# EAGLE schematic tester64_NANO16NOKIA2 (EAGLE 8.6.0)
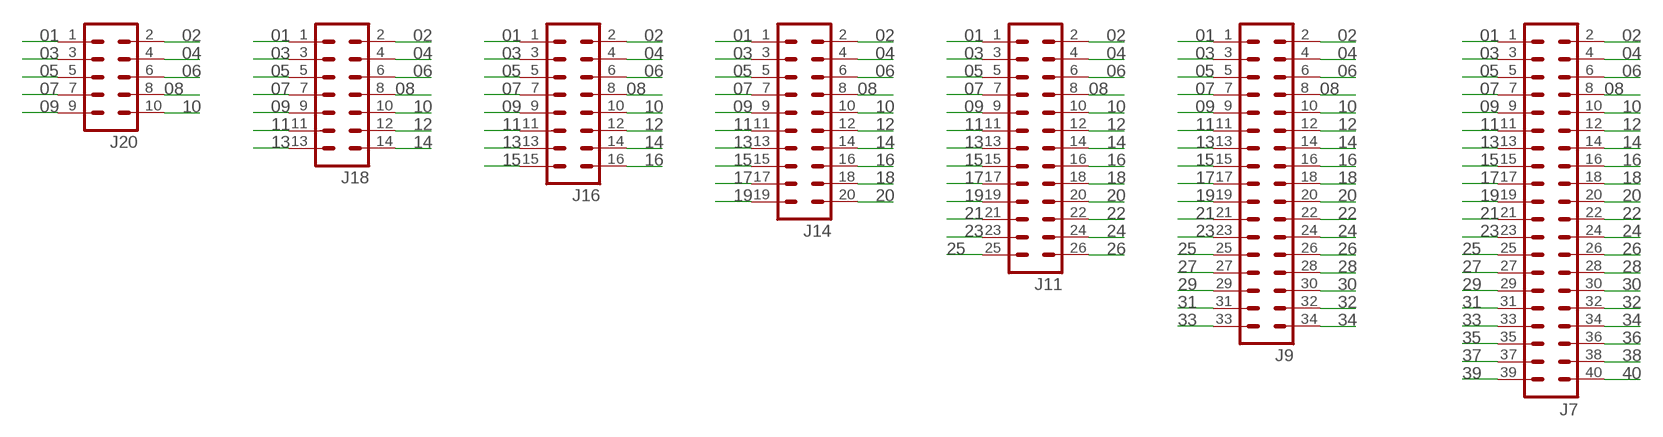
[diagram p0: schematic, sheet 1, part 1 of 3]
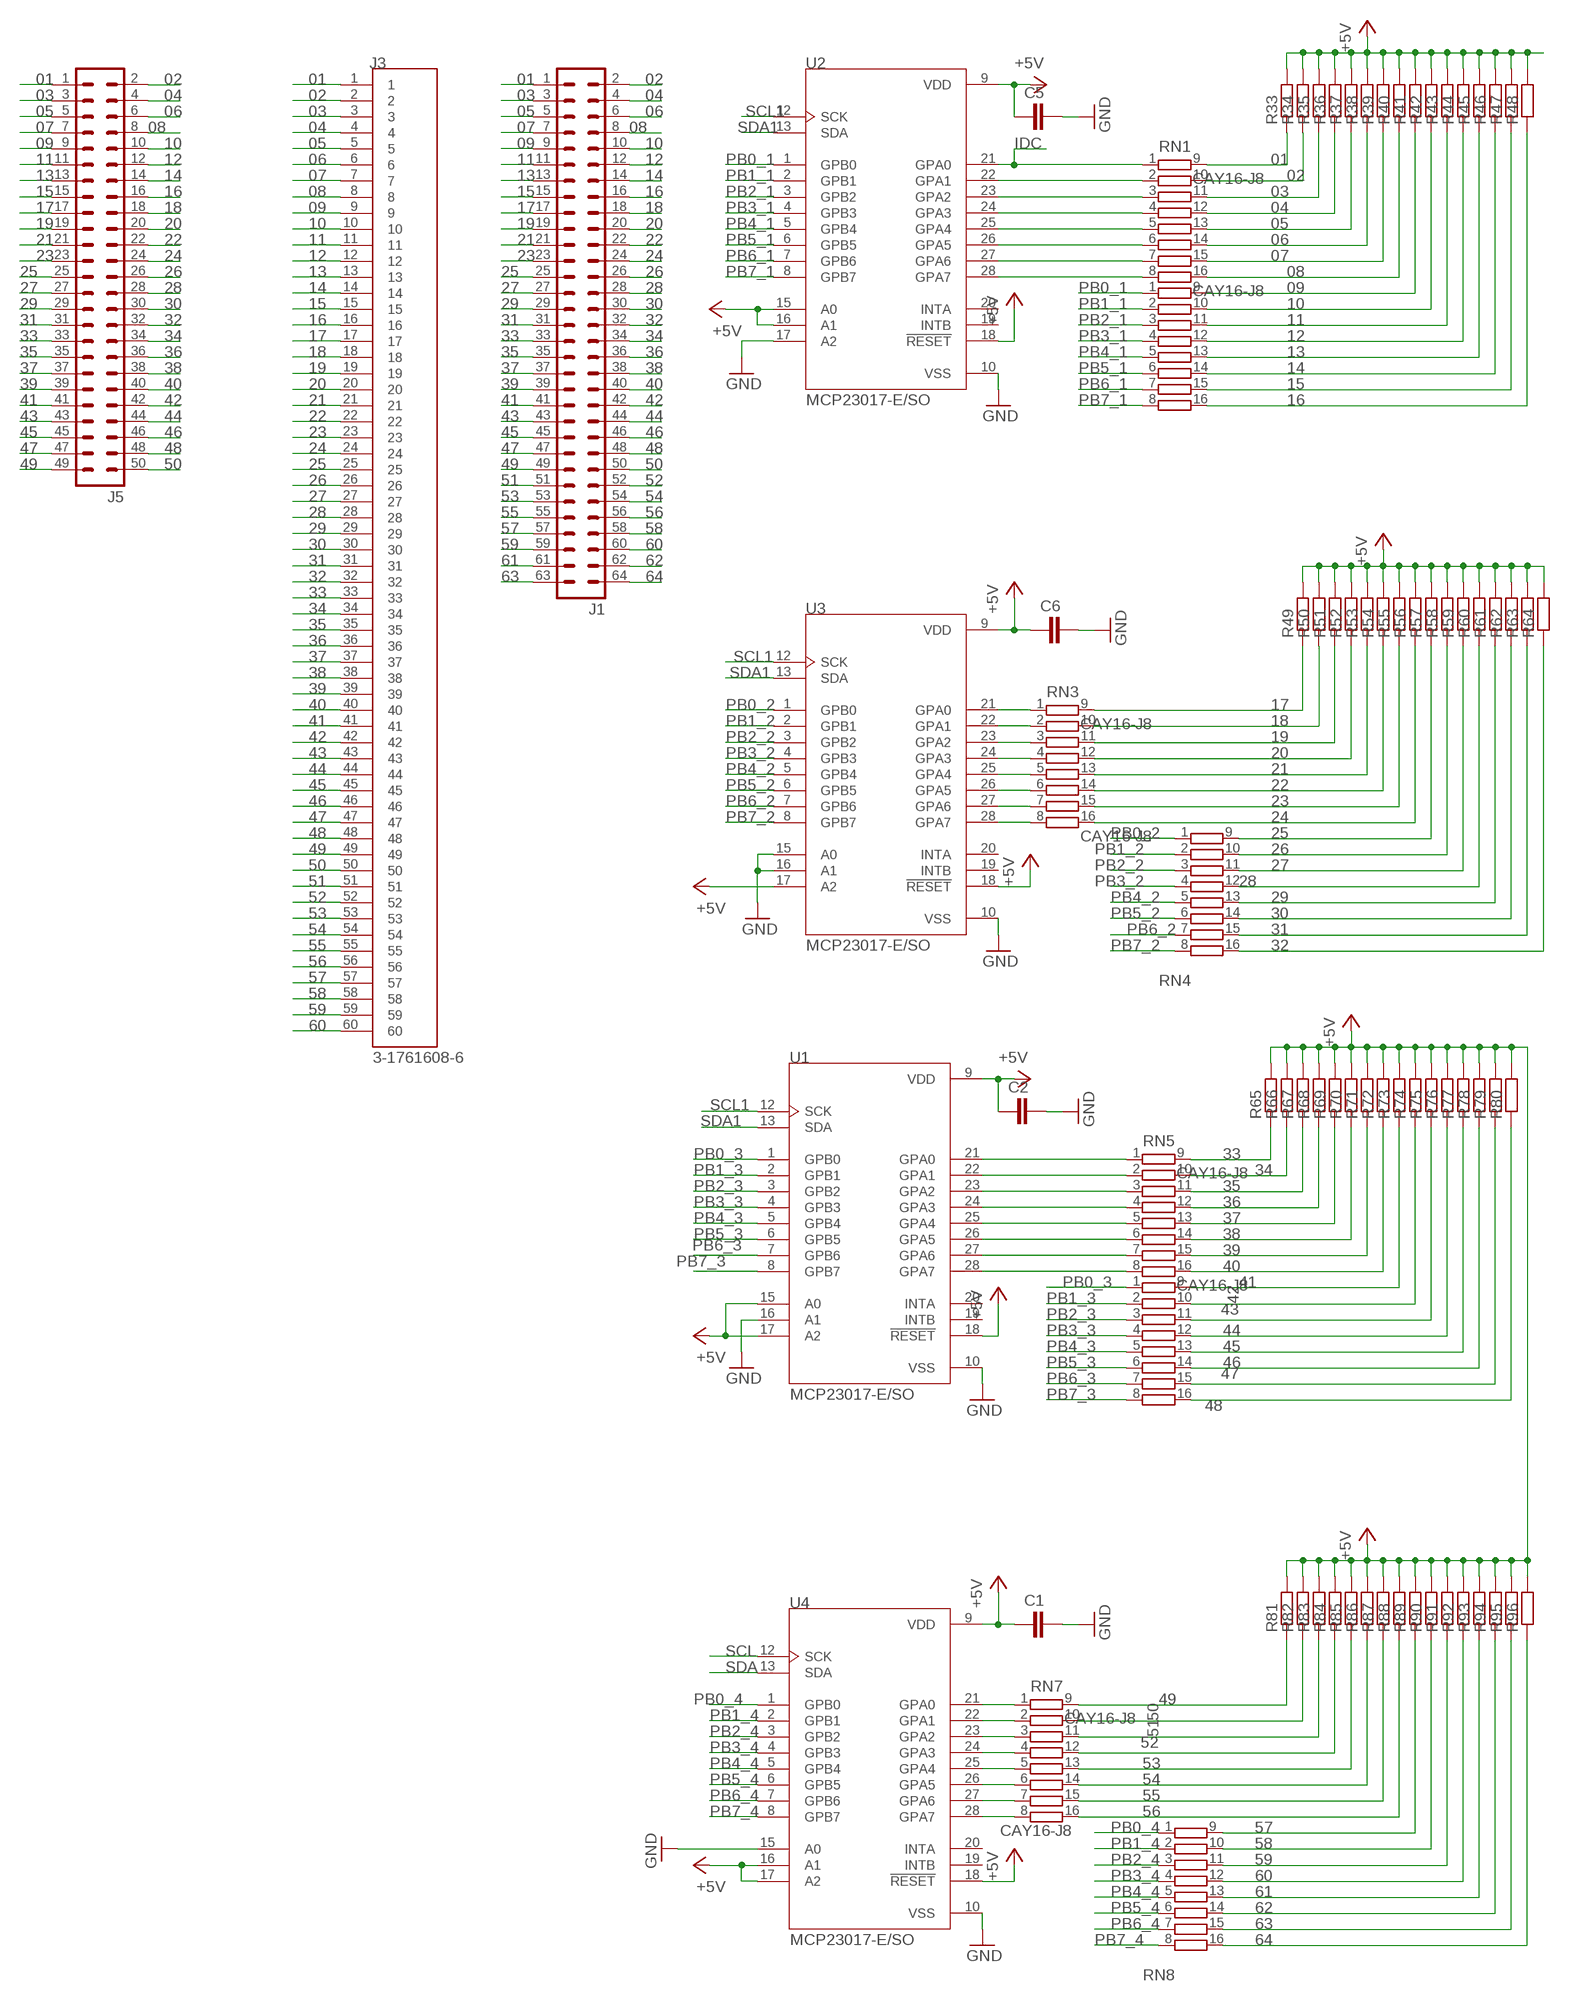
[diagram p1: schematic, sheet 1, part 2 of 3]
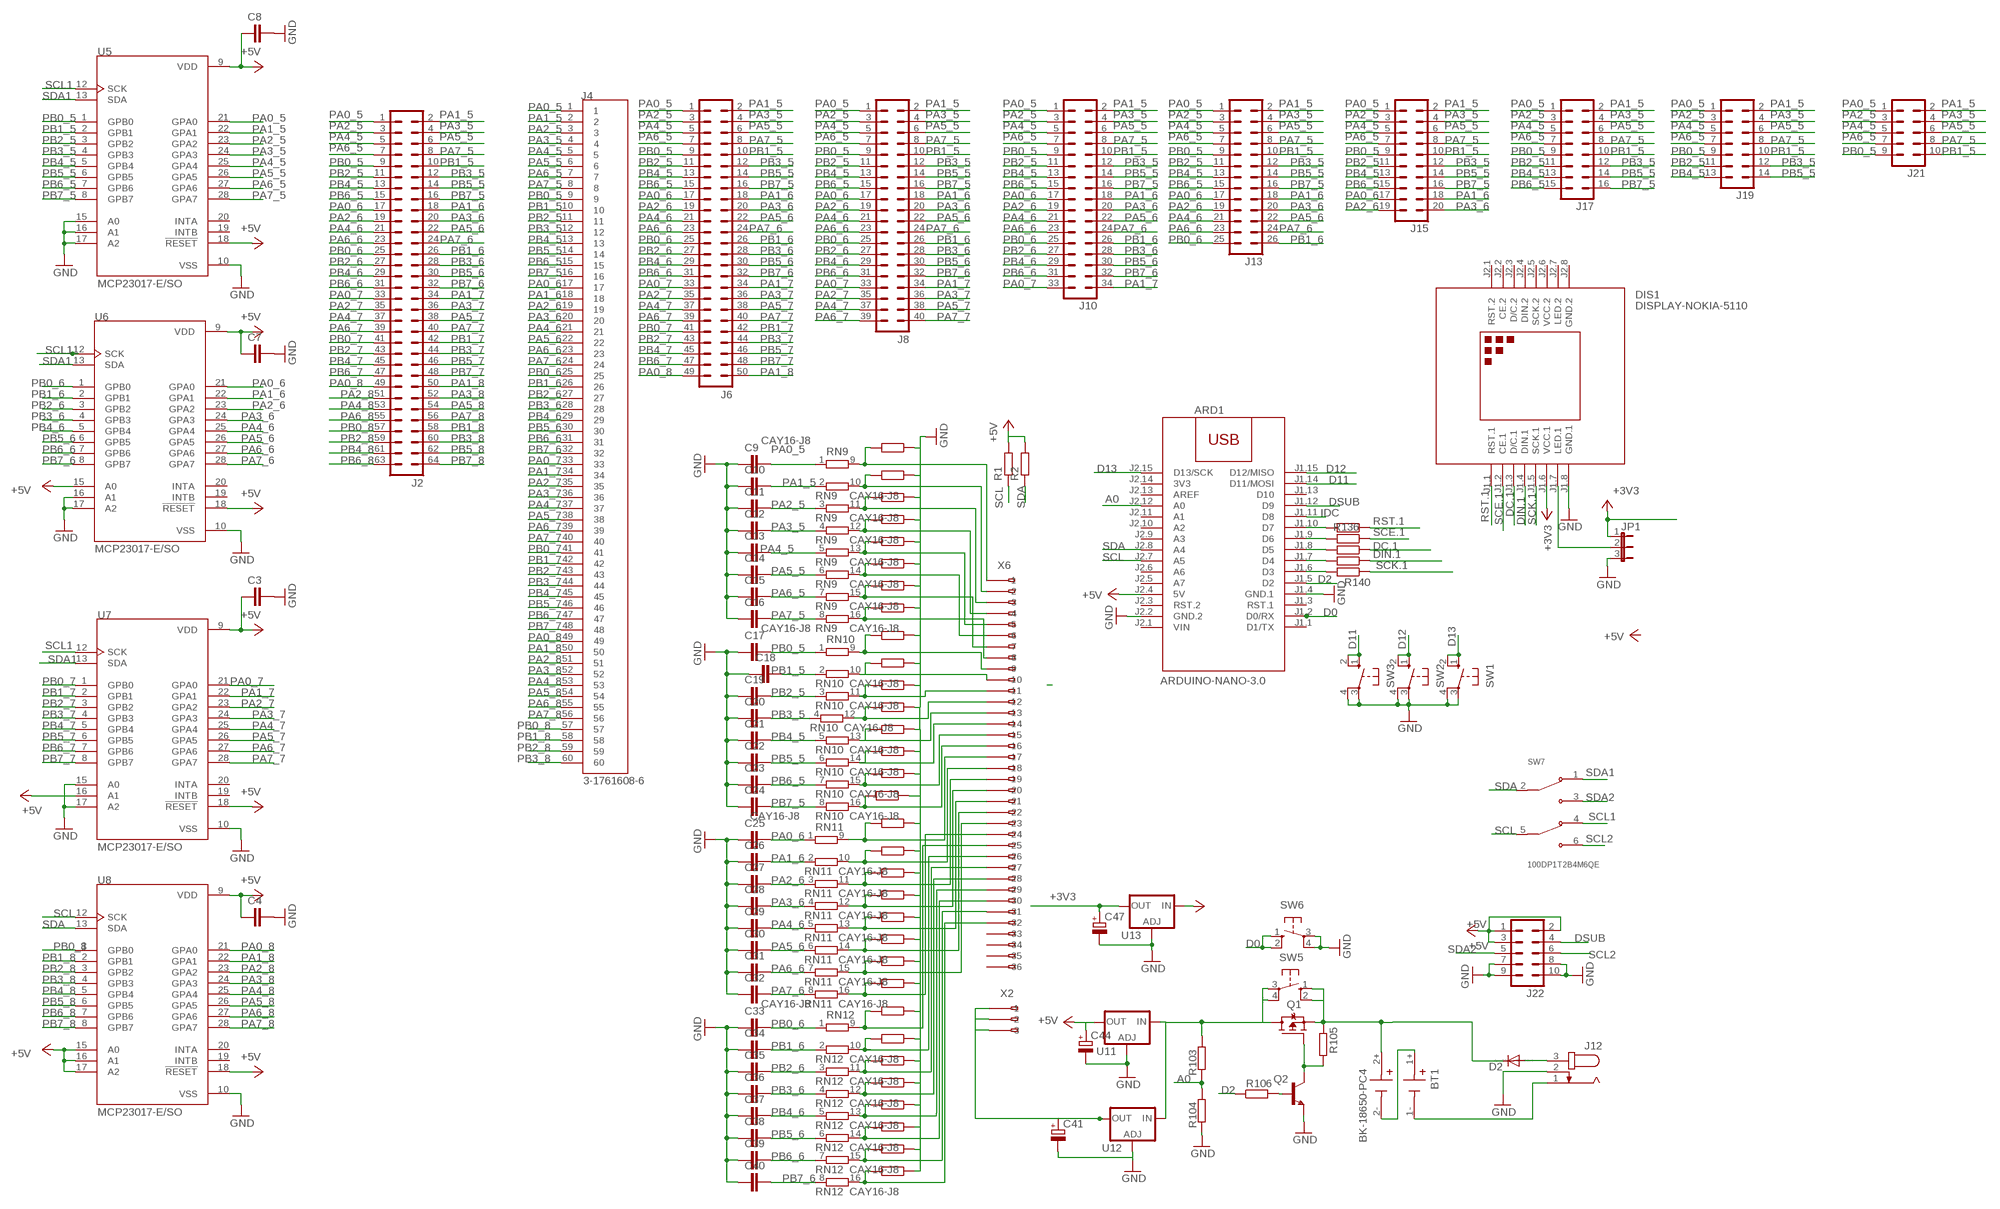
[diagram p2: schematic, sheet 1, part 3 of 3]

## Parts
ARD1  ARDUINO-NANO-3.0  [ARDUINO-NANO-3.0]
BT1  BK-18650-PC4  [BAT_BK-18650-PC4]
C1  C-EUC0603  [C0603]
C2  C-EUC0603  [C0603]
C3  C-EUC0603  [C0603]
C4  C-EUC0603  [C0603]
C5  C-EUC0603  [C0603]
C6  C-EUC0603  [C0603]
C7  C-EUC0603  [C0603]
C8  C-EUC0603  [C0603]
C9  C-EUC0603  [C0603]
C10  C-EUC0603  [C0603]
C11  C-EUC0603  [C0603]
C12  C-EUC0603  [C0603]
C13  C-EUC0603  [C0603]
C14  C-EUC0603  [C0603]
C15  C-EUC0603  [C0603]
C16  C-EUC0603  [C0603]
C17  C-EUC0603  [C0603]
C18  C-EUC0603  [C0603]
C19  C-EUC0603  [C0603]
C20  C-EUC0603  [C0603]
C21  C-EUC0603  [C0603]
C22  C-EUC0603  [C0603]
C23  C-EUC0603  [C0603]
C24  C-EUC0603  [C0603]
C25  C-EUC0603  [C0603]
C26  C-EUC0603  [C0603]
C27  C-EUC0603  [C0603]
C28  C-EUC0603  [C0603]
C29  C-EUC0603  [C0603]
C30  C-EUC0603  [C0603]
C31  C-EUC0603  [C0603]
C32  C-EUC0603  [C0603]
C33  C-EUC0603  [C0603]
C34  C-EUC0603  [C0603]
C35  C-EUC0603  [C0603]
C36  C-EUC0603  [C0603]
C37  C-EUC0603  [C0603]
C38  C-EUC0603  [C0603]
C39  C-EUC0603  [C0603]
C40  C-EUC0603  [C0603]
C41  CPOL-EUSMCB  [SMC_B]
C44  CPOL-EUSMCB  [SMC_B]
C47  CPOL-EUSMCB  [SMC_B]
D2  DIODE-SMB  [SMB]
DIS1  DISPLAY-NOKIA-5110  [DISPLAY-NOKIA-5110]
J1  ML64  [ML64]
J2  ML64  [ML64]
J3  3-1761608-6  [TE_3-1761608-6]
J4  3-1761608-6  [TE_3-1761608-6]
J5  ML50  [ML50]
J6  ML50  [ML50]
J7  ML40  [ML40]
J8  ML40  [ML40]
J9  ML34  [ML34]
J10  ML34  [ML34]
J11  ML26  [ML26]
J12  JACK-PLUG1  [SPC4078]
J13  ML26  [ML26]
J14  ML20  [ML20]
J15  ML20  [ML20]
J16  ML16  [ML16]
J17  ML16  [ML16]
J18  ML14  [ML14]
J19  ML14  [ML14]
J20  ML10  [ML10]
J21  ML10  [ML10]
J22  ML10  [ML10]
JP1  JP2E  [JP2]
Q1  STR2P3LLH6  [SOT23]
Q2  BC846  [SOT23]
R1  R-EU_R0805  [R0805]
R2  R-EU_R0805  [R0805]
R3  R-EU_R0805  [R0805]
R4  R-EU_R0805  [R0805]
R5  R-EU_R0805  [R0805]
R6  R-EU_R0805  [R0805]
R7  R-EU_R0805  [R0805]
R8  R-EU_R0805  [R0805]
R9  R-EU_R0805  [R0805]
R10  R-EU_R0805  [R0805]
R11  R-EU_R0805  [R0805]
R12  R-EU_R0805  [R0805]
R13  R-EU_R0805  [R0805]
R14  R-EU_R0805  [R0805]
R15  R-EU_R0805  [R0805]
R16  R-EU_R0805  [R0805]
R17  R-EU_R0805  [R0805]
R18  R-EU_R0805  [R0805]
R19  R-EU_R0805  [R0805]
R20  R-EU_R0805  [R0805]
R21  R-EU_R0805  [R0805]
R22  R-EU_R0805  [R0805]
R23  R-EU_R0805  [R0805]
R24  R-EU_R0805  [R0805]
R25  R-EU_R0805  [R0805]
R26  R-EU_R0805  [R0805]
R27  R-EU_R0805  [R0805]
R28  R-EU_R0805  [R0805]
R29  R-EU_R0805  [R0805]
R30  R-EU_R0805  [R0805]
R31  R-EU_R0805  [R0805]
R32  R-EU_R0805  [R0805]
R33  R-EU_R0402  [R0402]
R34  R-EU_R0402  [R0402]
R35  R-EU_R0402  [R0402]
R36  R-EU_R0402  [R0402]
R37  R-EU_R0402  [R0402]
R38  R-EU_R0402  [R0402]
R39  R-EU_R0402  [R0402]
R40  R-EU_R0402  [R0402]
R41  R-EU_R0402  [R0402]
R42  R-EU_R0402  [R0402]
R43  R-EU_R0402  [R0402]
R44  R-EU_R0402  [R0402]
R45  R-EU_R0402  [R0402]
R46  R-EU_R0402  [R0402]
R47  R-EU_R0402  [R0402]
R48  R-EU_R0402  [R0402]
R49  R-EU_R0402  [R0402]
R50  R-EU_R0402  [R0402]
R51  R-EU_R0402  [R0402]
R52  R-EU_R0402  [R0402]
R53  R-EU_R0402  [R0402]
R54  R-EU_R0402  [R0402]
R55  R-EU_R0402  [R0402]
R56  R-EU_R0402  [R0402]
R57  R-EU_R0402  [R0402]
R58  R-EU_R0402  [R0402]
R59  R-EU_R0402  [R0402]
R60  R-EU_R0402  [R0402]
R61  R-EU_R0402  [R0402]
R62  R-EU_R0402  [R0402]
R63  R-EU_R0402  [R0402]
R64  R-EU_R0402  [R0402]
R65  R-EU_R0402  [R0402]
R66  R-EU_R0402  [R0402]
R67  R-EU_R0402  [R0402]
R68  R-EU_R0402  [R0402]
R69  R-EU_R0402  [R0402]
R70  R-EU_R0402  [R0402]
R71  R-EU_R0402  [R0402]
R72  R-EU_R0402  [R0402]
R73  R-EU_R0402  [R0402]
R74  R-EU_R0402  [R0402]
R75  R-EU_R0402  [R0402]
R76  R-EU_R0402  [R0402]
R77  R-EU_R0402  [R0402]
R78  R-EU_R0402  [R0402]
R79  R-EU_R0402  [R0402]
R80  R-EU_R0402  [R0402]
R81  R-EU_R0402  [R0402]
R82  R-EU_R0402  [R0402]
R83  R-EU_R0402  [R0402]
R84  R-EU_R0402  [R0402]
R85  R-EU_R0402  [R0402]
R86  R-EU_R0402  [R0402]
R87  R-EU_R0402  [R0402]
R88  R-EU_R0402  [R0402]
R89  R-EU_R0402  [R0402]
R90  R-EU_R0402  [R0402]
R91  R-EU_R0402  [R0402]
R92  R-EU_R0402  [R0402]
R93  R-EU_R0402  [R0402]
R94  R-EU_R0402  [R0402]
R95  R-EU_R0402  [R0402]
R96  R-EU_R0402  [R0402]
R97  R-EU_R0805  [R0805]
R98  R-EU_R0805  [R0805]
R103  R-EU_R0805  [R0805]
R104  R-EU_R0805  [R0805]
R105  R-EU_R0805  [R0805]
R106  R-EU_R0805  [R0805]
R136  R-EU_R1206  [R1206]
R137  R-EU_R1206  [R1206]
R138  R-EU_R1206  [R1206]
R139  R-EU_R1206  [R1206]
R140  R-EU_R1206  [R1206]
RN1  CAY16-J8  [CAY16Y8]
RN2  CAY16-J8  [CAY16Y8]
RN3  CAY16-J8  [CAY16Y8]
RN4  CAY16-J8  [CAY16Y8]
RN5  CAY16-J8  [CAY16Y8]
RN6  CAY16-J8  [CAY16Y8]
RN7  CAY16-J8  [CAY16Y8]
RN8  CAY16-J8  [CAY16Y8]
RN9  CAY16-J8  [CAY16Y8]
RN10  CAY16-J8  [CAY16Y8]
RN11  CAY16-J8  [CAY16Y8]
RN12  CAY16-J8  [CAY16Y8]
SW1  10-XX  [B3F-10XX]
SW2  10-XX  [B3F-10XX]
SW3  10-XX  [B3F-10XX]
SW5  10-XX  [B3F-10XX]
SW6  10-XX  [B3F-10XX]
SW7  100DP1T2B4M6QE  [SW_100DP1T2B4M6QE]
U1  MCP23017-E/SO  [SOIC127P1030X265-28N]
U2  MCP23017-E/SO  [SOIC127P1030X265-28N]
U3  MCP23017-E/SO  [SOIC127P1030X265-28N]
U4  MCP23017-E/SO  [SOIC127P1030X265-28N]
U5  MCP23017-E/SO  [SOIC127P1030X265-28N]
U6  MCP23017-E/SO  [SOIC127P1030X265-28N]
U7  MCP23017-E/SO  [SOIC127P1030X265-28N]
U8  MCP23017-E/SO  [SOIC127P1030X265-28N]
U11  LD117ADT12TR  [DPACK]
U12  LD117ADT12TR  [DPACK]
U13  LD117ADT12TR  [DPACK]
X2  234-203  [234-203]
X6  234-236  [234-236]

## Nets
01: J1.1 J3.1 J5.1 J7.1 J9.1 J11.1 J14.1 J16.1 J18.1 J20.1 R33.1 RN1.9
02: J1.2 J3.2 J5.2 J7.2 J9.2 J11.2 J14.2 J16.2 J18.2 J20.2 R34.1 RN1.10
03: J1.3 J3.3 J5.3 J7.3 J9.3 J11.3 J14.3 J16.3 J18.3 J20.3 R35.1 RN1.11
04: J1.4 J3.4 J5.4 J7.4 J9.4 J11.4 J14.4 J16.4 J18.4 J20.4 R36.1 RN1.12
05: J1.5 J3.5 J5.5 J7.5 J9.5 J11.5 J14.5 J16.5 J18.5 J20.5 R37.1 RN1.13
06: J1.6 J3.6 J5.6 J7.6 J9.6 J11.6 J14.6 J16.6 J18.6 J20.6 R38.1 RN1.14
07: J1.7 J3.7 J5.7 J7.7 J9.7 J11.7 J14.7 J16.7 J18.7 J20.7 R39.1 RN1.15
08: J1.8 J3.8 J5.8 J7.8 J9.8 J11.8 J14.8 J16.8 J18.8 J20.8 R40.1 RN1.16
09: J1.9 J3.9 J5.9 J7.9 J9.9 J11.9 J14.9 J16.9 J18.9 J20.9 R41.1 RN2.9
10: J1.10 J3.10 J5.10 J7.10 J9.10 J11.10 J14.10 J16.10 J18.10 J20.10 R42.1 RN2.10
11: J1.11 J3.11 J5.11 J7.11 J9.11 J11.11 J14.11 J16.11 J18.11 R43.1 RN2.11
12: J1.12 J3.12 J5.12 J7.12 J9.12 J11.12 J14.12 J16.12 J18.12 R44.1 RN2.12
13: J1.13 J3.13 J5.13 J7.13 J9.13 J11.13 J14.13 J16.13 J18.13 R45.1 RN2.13
14: J1.14 J3.14 J5.14 J7.14 J9.14 J11.14 J14.14 J16.14 J18.14 R46.1 RN2.14
15: J1.15 J3.15 J5.15 J7.15 J9.15 J11.15 J14.15 J16.15 R47.1 RN2.15
16: J1.16 J3.16 J5.16 J7.16 J9.16 J11.16 J14.16 J16.16 R48.1 RN2.16
17: J1.17 J3.17 J5.17 J7.17 J9.17 J11.17 J14.17 R49.1 RN3.9
18: J1.18 J3.18 J5.18 J7.18 J9.18 J11.18 J14.18 R50.1 RN3.10
19: J1.19 J3.19 J5.19 J7.19 J9.19 J11.19 J14.19 R51.1 RN3.11
20: J1.20 J3.20 J5.20 J7.20 J9.20 J11.20 J14.20 R52.1 RN3.12
21: J1.21 J3.21 J5.21 J7.21 J9.21 J11.21 R53.1 RN3.13
22: J1.22 J3.22 J5.22 J7.22 J9.22 J11.22 R54.1 RN3.14
23: J1.23 J3.23 J5.23 J7.23 J9.23 J11.23 R55.1 RN3.15
24: J1.24 J3.24 J5.24 J7.24 J9.24 J11.24 R56.1 RN3.16
25: J1.25 J3.25 J5.25 J7.25 J9.25 J11.25 R57.1 RN4.9
26: J1.26 J3.26 J5.26 J7.26 J9.26 J11.26 R58.1 RN4.10
27: J1.27 J3.27 J5.27 J7.27 J9.27 R59.1 RN4.11
28: J1.28 J3.28 J5.28 J7.28 J9.28 R60.1 RN4.12
29: J1.29 J3.29 J5.29 J7.29 J9.29 R61.1 RN4.13
30: J1.30 J3.30 J5.30 J7.30 J9.30 R62.1 RN4.14
31: J1.31 J3.31 J5.31 J7.31 J9.31 R63.1 RN4.15
32: J1.32 J3.32 J5.32 J7.32 J9.32 R64.1 RN4.16
33: J1.33 J3.33 J5.33 J7.33 J9.33 R65.1 RN5.9
34: J1.34 J3.34 J5.34 J7.34 J9.34 R66.1 RN5.10
35: J1.35 J3.35 J5.35 J7.35 R67.1 RN5.11
36: J1.36 J3.36 J5.36 J7.36 R68.1 RN5.12
37: J1.37 J3.37 J5.37 J7.37 R69.1 RN5.13
38: J1.38 J3.38 J5.38 J7.38 R70.1 RN5.14
39: J1.39 J3.39 J5.39 J7.39 R71.1 RN5.15
40: J1.40 J3.40 J5.40 J7.40 R72.1 RN5.16
41: J1.41 J3.41 J5.41 R73.1 RN6.9
42: J1.42 J3.42 J5.42 R74.1 RN6.10
43: J1.43 J3.43 J5.43 R75.1 RN6.11
44: J1.44 J3.44 J5.44 R76.1 RN6.12
45: J1.45 J3.45 J5.45 R77.1 RN6.13
46: J1.46 J3.46 J5.46 R78.1 RN6.14
47: J1.47 J3.47 J5.47 R79.1 RN6.15
48: J1.48 J3.48 J5.48 R80.1 RN6.16
49: J1.49 J3.49 J5.49 R81.1 RN7.9
50: J1.50 J3.50 J5.50 R82.1 RN7.10
51: J1.51 J3.51 R83.1 RN7.11
52: J1.52 J3.52 R84.1 RN7.12
53: J1.53 J3.53 R85.1 RN7.13
54: J1.54 J3.54 R86.1 RN7.14
55: J1.55 J3.55 R87.1 RN7.15
56: J1.56 J3.56 R88.1 RN7.16
57: J1.57 J3.57 R89.1 RN8.9
58: J1.58 J3.58 R90.1 RN8.10
59: J1.59 J3.59 R91.1 RN8.11
60: J1.60 J3.60 R92.1 RN8.12
61: J1.61 R93.1 RN8.13
62: J1.62 R94.1 RN8.14
63: J1.63 R95.1 RN8.15
64: J1.64 R96.1 RN8.16
+3V3: C47.+ DIS1.J1.6(VCC.1) JP1.1 U13.4(OUT)
+5V: ARD1.J2.4(5V) C1.2 C2.2 C3.2 C4.2 C5.2 C6.2 C7.2 C8.2 C44.+ J22.1 J22.2 J22.3 R1.2 R2.2 R33.2 R34.2 R35.2 R36.2 R37.2 R38.2 R39.2 R40.2 R41.2 R42.2 R43.2 R44.2 R45.2 R46.2 R47.2 R48.2 R49.2 R50.2 R51.2 R52.2 R53.2 R54.2 R55.2 R56.2 R57.2 R58.2 R59.2 R60.2 R61.2 R62.2 R63.2 R64.2 R65.2 R66.2 R67.2 R68.2 R69.2 R70.2 R71.2 R72.2 R73.2 R74.2 R75.2 R76.2 R77.2 R78.2 R79.2 R80.2 R81.2 R82.2 R83.2 R84.2 R85.2 R86.2 R87.2 R88.2 R89.2 R90.2 R91.2 R92.2 R93.2 R94.2 R95.2 R96.2 U1.9(VDD) U1.15(A0) U1.17(A2) U1.18(!RESET) U2.9(VDD) U2.15(A0) U2.16(A1) U2.18(!RESET) U3.9(VDD) U3.17(A2) U3.18(!RESET) U4.9(VDD) U4.16(A1) U4.17(A2) U4.18(!RESET) U5.9(VDD) U5.18(!RESET) U6.9(VDD) U6.15(A0) U6.18(!RESET) U7.9(VDD) U7.16(A1) U7.18(!RESET) U8.9(VDD) U8.15(A0) U8.16(A1) U8.17(A2) U8.18(!RESET) U11.4(OUT) U13.3(IN)
A0: ARD1.J2.12(A0) R103.2 R104.1
D0: ARD1.J1.2(D0/RX) SW6.1(S) SW6.2(S1)
D2: ARD1.J1.5(D2) R106.1
D11: ARD1.J1.14(D11/MOSI) SW3.1(S) SW3.2(S1)
D12: ARD1.J1.15(D12/MISO) SW2.1(S) SW2.2(S1)
D13: ARD1.J2.15(D13/SCK) SW1.1(S) SW1.2(S1)
DC.1: DIS1.J1.3(D/C.1) R138.1
DIN.1: DIS1.J1.4(DIN.1) R139.1
DSUB: ARD1.J1.12(D9) J22.4
GND: ARD1.J1.4(GND.1) ARD1.J2.2(GND.2) C1.1 C2.1 C3.1 C4.1 C5.1 C6.1 C7.1 C8.1 C9.2 C10.2 C11.2 C12.2 C13.2 C14.2 C15.2 C16.2 C17.2 C18.2 C19.2 C20.2 C21.2 C22.2 C23.2 C24.2 C25.2 C26.2 C27.2 C28.2 C29.2 C30.2 C31.2 C32.2 C33.2 C34.2 C35.2 C36.2 C37.2 C38.2 C39.2 C40.2 C41.- C44.- C47.- DIS1.J1.8(GND.1) J12.2 J22.7 J22.8 J22.9 J22.10 JP1.3 Q2.2(E) R3.1 R4.1 R5.1 R6.1 R7.1 R8.1 R9.1 R10.1 R11.1 R12.1 R13.1 R14.1 R15.1 R16.1 R17.1 R18.1 R19.1 R20.1 R21.1 R22.1 R23.1 R24.1 R25.1 R26.1 R27.1 R28.1 R29.1 R30.1 R31.1 R32.1 R97.1 R98.1 R104.2 SW1.3(P) SW1.4(P1) SW2.3(P) SW2.4(P1) SW3.3(P) SW3.4(P1) SW6.3(P) SW6.4(P1) U1.10(VSS) U1.16(A1) U2.10(VSS) U2.17(A2) U3.10(VSS) U3.15(A0) U3.16(A1) U4.10(VSS) U4.15(A0) U5.10(VSS) U5.15(A0) U5.16(A1) U5.17(A2) U6.10(VSS) U6.16(A1) U6.17(A2) U7.10(VSS) U7.15(A0) U7.17(A2) U8.10(VSS) U11.1(ADJ) U12.1(ADJ) U13.1(ADJ)
IDC: ARD1.J1.11(D8) RN1.1 U2.21(GPA0)
N$2: RN1.2 U2.22(GPA1)
N$3: RN1.3 U2.23(GPA2)
N$4: RN1.4 U2.24(GPA3)
N$5: RN1.5 U2.25(GPA4)
N$6: RN1.6 U2.26(GPA5)
N$7: RN1.7 U2.27(GPA6)
N$8: RN1.8 U2.28(GPA7)
N$9: RN3.1 U3.21(GPA0)
N$10: RN3.2 U3.22(GPA1)
N$11: RN3.3 U3.23(GPA2)
N$12: RN3.4 U3.24(GPA3)
N$13: RN3.5 U3.25(GPA4)
N$14: RN3.6 U3.26(GPA5)
N$15: RN3.7 U3.27(GPA6)
N$16: RN3.8 U3.28(GPA7)
N$17: R3.2 RN9.9 X6.A1(-1)
N$18: R4.2 RN9.10 X6.A2(-2)
N$19: R5.2 RN9.11 X6.A3(-3)
N$20: R6.2 RN9.12 X6.A4(-4)
N$21: R7.2 RN9.13 X6.A5(-5)
N$22: R8.2 RN9.14 X6.A6(-6)
N$23: BT1.2+ D2.C Q1.3(S) R105.1 SW5.1(S) SW5.2(S1)
N$25: D2.A J12.3
N$26: R9.2 RN9.15 X6.A7(-7)
N$27: R10.2 RN9.16 X6.A8(-8)
N$28: RN5.1 U1.21(GPA0)
N$29: R16.2 RN10.14 X6.A14(-14)
N$30: RN5.2 U1.22(GPA1)
N$31: RN5.3 U1.23(GPA2)
N$32: RN5.4 U1.24(GPA3)
N$33: RN5.5 U1.25(GPA4)
N$34: RN5.6 U1.26(GPA5)
N$35: RN5.7 U1.27(GPA6)
N$36: RN5.8 U1.28(GPA7)
N$37: RN7.1 U4.21(GPA0)
N$38: RN7.2 U4.22(GPA1)
N$39: RN7.3 U4.23(GPA2)
N$40: RN7.4 U4.24(GPA3)
N$41: RN7.5 U4.25(GPA4)
N$42: RN7.6 U4.26(GPA5)
N$43: RN7.7 U4.27(GPA6)
N$44: RN7.8 U4.28(GPA7)
N$45: R12.2 RN10.10 X6.A10(-10)
N$46: R15.2 RN10.13 X6.A13(-13)
N$47: R13.2 RN10.11 X6.A11(-11)
N$48: R17.2 RN10.15 X6.A15(-15)
N$49: C41.+ U12.4(OUT) X2.A1(-1) X2.A2(-2) X2.A3(-3)
N$50: R19.2 RN11.9 X6.A17(-17)
N$51: R23.2 RN11.13 X6.A21(-21)
N$52: R18.2 RN10.16 X6.A16(-16)
N$53: R25.2 RN11.15 X6.A23(-23)
N$54: R26.2 RN11.16 X6.A24(-24)
N$55: R27.2 RN12.9 X6.A25(-25)
N$56: R28.2 RN12.10 X6.A26(-26)
N$58: R29.2 RN12.11 X6.A27(-27)
N$59: Q1.2(G) Q2.3(C) R105.2
N$60: R31.2 RN12.13 X6.A29(-29)
N$61: BT1.1+ BT1.2-
N$62: BT1.1- J12.1
N$63: R11.2 RN10.9 X6.A9(-9)
N$64: ARD1.J1.10(D7) R136.2
N$65: R30.2 RN12.12 X6.A28(-28)
N$66: ARD1.J1.9(D6) R137.2
N$67: R32.2 RN12.14 X6.A30(-30)
N$68: ARD1.J1.8(D5) R138.2
N$69: ARD1.J1.7(D4) R139.2
N$71: ARD1.J1.6(D3) R140.2
N$72: DIS1.J1.7(LED.1) JP1.2
N$81: R14.2 RN10.12 X6.A12(-12)
N$87: R20.2 RN11.10 X6.A18(-18)
N$88: R21.2 RN11.11 X6.A19(-19)
N$89: R22.2 RN11.12 X6.A20(-20)
N$91: R24.2 RN11.14 X6.A22(-22)
N$107: R97.2 RN12.15 X6.A31(-31)
N$108: R98.2 RN12.16 X6.A32(-32)
N$112: Q1.1(D) R103.1 SW5.3(P) SW5.4(P1) U11.3(IN) U12.3(IN)
N$114: Q2.1(B) R106.2
PA0_5: C9.1 J2.1 J4.1 J6.1 J8.1 J10.1 J13.1 J15.1 J17.1 J19.1 J21.1 RN9.1 U5.21(GPA0)
PA0_6: C25.1 J2.17 J4.17 J6.17 J8.17 J10.17 J13.17 J15.17 RN11.1 U6.21(GPA0)
PA0_7: J2.33 J4.33 J6.33 J8.33 J10.33 U7.21(GPA0)
PA0_8: J2.49 J4.49 J6.49 U8.21(GPA0)
PA1_5: C10.1 J2.2 J4.2 J6.2 J8.2 J10.2 J13.2 J15.2 J17.2 J19.2 J21.2 RN9.2 U5.22(GPA1)
PA1_6: C26.1 J2.18 J4.18 J6.18 J8.18 J10.18 J13.18 J15.18 RN11.2 U6.22(GPA1)
PA1_7: J2.34 J4.34 J6.34 J8.34 J10.34 U7.22(GPA1)
PA1_8: J2.50 J4.50 J6.50 U8.22(GPA1)
PA2_5: C11.1 J2.3 J4.3 J6.3 J8.3 J10.3 J13.3 J15.3 J17.3 J19.3 J21.3 RN9.3 U5.23(GPA2)
PA2_6: C27.1 J2.19 J4.19 J6.19 J8.19 J10.19 J13.19 J15.19 RN11.3 U6.23(GPA2)
PA2_7: J2.35 J4.35 J6.35 J8.35 U7.23(GPA2)
PA2_8: J2.51 J4.51 U8.23(GPA2)
PA3_5: C12.1 J2.4 J4.4 J6.4 J8.4 J10.4 J13.4 J15.4 J17.4 J19.4 J21.4 RN9.4 U5.24(GPA3)
PA3_6: C28.1 J2.20 J4.20 J6.20 J8.20 J10.20 J13.20 J15.20 RN11.4 U6.24(GPA3)
PA3_7: J2.36 J4.36 J6.36 J8.36 U7.24(GPA3)
PA3_8: J2.52 J4.52 U8.24(GPA3)
PA4_5: C13.1 J2.5 J4.5 J6.5 J8.5 J10.5 J13.5 J15.5 J17.5 J19.5 J21.5 RN9.5 U5.25(GPA4)
PA4_6: C29.1 J2.21 J4.21 J6.21 J8.21 J10.21 J13.21 RN11.5 U6.25(GPA4)
PA4_7: J2.37 J4.37 J6.37 J8.37 U7.25(GPA4)
PA4_8: J2.53 J4.53 U8.25(GPA4)
PA5_5: C14.1 J2.6 J4.6 J6.6 J8.6 J10.6 J13.6 J15.6 J17.6 J19.6 J21.6 RN9.6 U5.26(GPA5)
PA5_6: C30.1 J2.22 J4.22 J6.22 J8.22 J10.22 J13.22 RN11.6 U6.26(GPA5)
PA5_7: J2.38 J4.38 J6.38 J8.38 U7.26(GPA5)
PA5_8: J2.54 J4.54 U8.26(GPA5)
PA6_5: C15.1 J2.7 J4.7 J6.7 J8.7 J10.7 J13.7 J15.7 J17.7 J19.7 J21.7 RN9.7 U5.27(GPA6)
PA6_6: C31.1 J2.23 J4.23 J6.23 J8.23 J10.23 J13.23 RN11.7 U6.27(GPA6)
PA6_7: J2.39 J4.39 J6.39 J8.39 U7.27(GPA6)
PA6_8: J2.55 J4.55 U8.27(GPA6)
PA7_5: C16.1 J2.8 J4.8 J6.8 J8.8 J10.8 J13.8 J15.8 J17.8 J19.8 J21.8 RN9.8 U5.28(GPA7)
PA7_6: C32.1 J2.24 J4.24 J6.24 J8.24 J10.24 J13.24 RN11.8 U6.28(GPA7)
PA7_7: J2.40 J4.40 J6.40 J8.40 U7.28(GPA7)
PA7_8: J2.56 J4.56 U8.28(GPA7)
PB0_1: RN2.1 U2.1(GPB0)
PB0_2: RN4.1 U3.1(GPB0)
PB0_3: RN6.1 U1.1(GPB0)
PB0_4: RN8.1 U4.1(GPB0)
PB0_5: C17.1 J2.9 J4.9 J6.9 J8.9 J10.9 J13.9 J15.9 J17.9 J19.9 J21.9 RN10.1 U5.1(GPB0)
PB0_6: C33.1 J2.25 J4.25 J6.25 J8.25 J10.25 J13.25 RN12.1 U6.1(GPB0)
PB0_7: J2.41 J4.41 J6.41 U7.1(GPB0)
PB0_8: J2.57 J4.57 U8.1(GPB0)
PB1_1: RN2.2 U2.2(GPB1)
PB1_2: RN4.2 U3.2(GPB1)
PB1_3: RN6.2 U1.2(GPB1)
PB1_4: RN8.2 U4.2(GPB1)
PB1_5: C18.1 J2.10 J4.10 J6.10 J8.10 J10.10 J13.10 J15.10 J17.10 J19.10 J21.10 RN10.2 U5.2(GPB1)
PB1_6: C34.1 J2.26 J4.26 J6.26 J8.26 J10.26 J13.26 RN12.2 U6.2(GPB1)
PB1_7: J2.42 J4.42 J6.42 U7.2(GPB1)
PB1_8: J2.58 J4.58 U8.2(GPB1)
PB2_1: RN2.3 U2.3(GPB2)
PB2_2: RN4.3 U3.3(GPB2)
PB2_3: RN6.3 U1.3(GPB2)
PB2_4: RN8.3 U4.3(GPB2)
PB2_5: C19.1 J2.11 J4.11 J6.11 J8.11 J10.11 J13.11 J15.11 J17.11 J19.11 RN10.3 U5.3(GPB2)
PB2_6: C35.1 J2.27 J4.27 J6.27 J8.27 J10.27 RN12.3 U6.3(GPB2)
PB2_7: J2.43 J4.43 J6.43 U7.3(GPB2)
PB2_8: J2.59 J4.59 U8.3(GPB2)
PB3_1: RN2.4 U2.4(GPB3)
PB3_2: RN4.4 U3.4(GPB3)
PB3_3: RN6.4 U1.4(GPB3)
PB3_4: RN8.4 U4.4(GPB3)
PB3_5: C20.1 J2.12 J4.12 J6.12 J8.12 J10.12 J13.12 J15.12 J17.12 J19.12 RN10.4 U5.4(GPB3)
PB3_6: C36.1 J2.28 J4.28 J6.28 J8.28 J10.28 RN12.4 U6.4(GPB3)
PB3_7: J2.44 J4.44 J6.44 U7.4(GPB3)
PB3_8: J2.60 J4.60 U8.4(GPB3)
PB4_1: RN2.5 U2.5(GPB4)
PB4_2: RN4.5 U3.5(GPB4)
PB4_3: RN6.5 U1.5(GPB4)
PB4_4: RN8.5 U4.5(GPB4)
PB4_5: C21.1 J2.13 J4.13 J6.13 J8.13 J10.13 J13.13 J15.13 J17.13 J19.13 RN10.5 U5.5(GPB4)
PB4_6: C37.1 J2.29 J4.29 J6.29 J8.29 J10.29 RN12.5 U6.5(GPB4)
PB4_7: J2.45 J4.45 J6.45 U7.5(GPB4)
PB4_8: J2.61 U8.5(GPB4)
PB5_1: RN2.6 U2.6(GPB5)
PB5_2: RN4.6 U3.6(GPB5)
PB5_3: RN6.6 U1.6(GPB5)
PB5_4: RN8.6 U4.6(GPB5)
PB5_5: C22.1 J2.14 J4.14 J6.14 J8.14 J10.14 J13.14 J15.14 J17.14 J19.14 RN10.6 U5.6(GPB5)
PB5_6: C38.1 J2.30 J4.30 J6.30 J8.30 J10.30 RN12.6 U6.6(GPB5)
PB5_7: J2.46 J4.46 J6.46 U7.6(GPB5)
PB5_8: J2.62 U8.6(GPB5)
PB6_1: RN2.7 U2.7(GPB6)
PB6_2: RN4.7 U3.7(GPB6)
PB6_3: RN6.7 U1.7(GPB6)
PB6_4: RN8.7 U4.7(GPB6)
PB6_5: C23.1 J2.15 J4.15 J6.15 J8.15 J10.15 J13.15 J15.15 J17.15 RN10.7 U5.7(GPB6)
PB6_6: C39.1 J2.31 J4.31 J6.31 J8.31 J10.31 RN12.7 U6.7(GPB6)
PB6_7: J2.47 J4.47 J6.47 U7.7(GPB6)
PB6_8: J2.63 U8.7(GPB6)
PB7_1: RN2.8 U2.8(GPB7)
PB7_2: RN4.8 U3.8(GPB7)
PB7_3: RN6.8 U1.8(GPB7)
PB7_4: RN8.8 U4.8(GPB7)
PB7_5: C24.1 J2.16 J4.16 J6.16 J8.16 J10.16 J13.16 J15.16 J17.16 RN10.8 U5.8(GPB7)
PB7_6: C40.1 J2.32 J4.32 J6.32 J8.32 J10.32 RN12.8 U6.8(GPB7)
PB7_7: J2.48 J4.48 J6.48 U7.8(GPB7)
PB7_8: J2.64 U8.8(GPB7)
RST.1: DIS1.J1.1(RST.1) R136.1
SCE.1: DIS1.J1.2(CE.1) R137.1
SCK.1: DIS1.J1.5(SCK.1) R140.1
SCL: ARD1.J2.7(A5) R1.1 SW7.5 U4.12(SCK) U8.12(SCK)
SCL1: SW7.4 U1.12(SCK) U2.12(SCK) U3.12(SCK) U5.12(SCK) U6.12(SCK) U7.12(SCK)
SCL2: J22.6 SW7.6
SDA: ARD1.J2.8(A4) R2.1 SW7.2 U4.13(SDA) U8.13(SDA)
SDA1: SW7.1 U1.13(SDA) U2.13(SDA) U3.13(SDA) U5.13(SDA) U6.13(SDA) U7.13(SDA)
SDA2: J22.5 SW7.3
Unconnected: ARD1.J1.1(D1/TX) ARD1.J1.3(RST.1) ARD1.J1.13(D10) ARD1.J2.3(RST.2) ARD1.J2.5(A7) ARD1.J2.6(A6) ARD1.J2.9(A3) ARD1.J2.10(A2) ARD1.J2.11(A1) ARD1.J2.13(AREF) DIS1.J2.1(RST.2) DIS1.J2.2(CE.2) DIS1.J2.3(D/C.2) DIS1.J2.4(DIN.2) DIS1.J2.5(SCK.2) DIS1.J2.7(LED.2) U1.19(INTB) U1.20(INTA) U2.19(INTB) U2.20(INTA) U3.19(INTB) U3.20(INTA) U4.19(INTB) U4.20(INTA) U5.19(INTB) U5.20(INTA) U6.19(INTB) U6.20(INTA) U7.19(INTB) U7.20(INTA) U8.19(INTB) U8.20(INTA) X2.B1(B-1) X2.B2(B-2) X2.B3(B-3) X6.A33(-33) X6.A34(-34) X6.A35(-35) X6.A36(-36) X6.B1(B-1) X6.B2(B-2) X6.B3(B-3) X6.B4(B-4) X6.B5(B-5) X6.B6(B-6) X6.B7(B-7) X6.B8(B-8) X6.B9(B-9) X6.B10(B-10) X6.B11(B-11) X6.B12(B-12) X6.B13(B-13) X6.B14(B-14) X6.B15(B-15) X6.B16(B-16) X6.B17(B-17) X6.B18(B-18) X6.B19(B-19) X6.B20(B-20) X6.B21(B-21) X6.B22(B-22) X6.B23(B-23) X6.B24(B-24) X6.B25(B-25) X6.B26(B-26) X6.B27(B-27) X6.B28(B-28) X6.B29(B-29) X6.B30(B-30) X6.B31(B-31) X6.B32(B-32) X6.B33(B-33) X6.B34(B-34) X6.B35(B-35) X6.B36(B-36)

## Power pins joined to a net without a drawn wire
3V3: ARD1.J2.14(3V3)
GND.2: DIS1.J2.8(GND.2)
VCC.2: DIS1.J2.6(VCC.2)
VIN: ARD1.J2.1(VIN)

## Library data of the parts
ARD1 = diy-modules:ARDUINO-NANO-3.0: Arduino Nano 3.0 and compatible devices More details available here: https://www.arduino.cc/en/Main/ArduinoBoardNano Click here to find device on ebay.com
BT1 = BK-18650-PC4:BK-18650-PC4: Battery Holder (Open) 18650 2 Cell PC Pin Check availability; AVAILABILITY: In Stock; CHECK_PRICES: https://www.snapeda.com/parts/BK-18650-PC4/Memory+Protection+Devices/view-part/?ref=eda; DESCRIPTION: Battery Holder (Open) 18650 2 Cell PC Pin; MF: MPD (Memory Protection Devices); MP: BK-18650-PC4; PACKAGE: None; PRICE: None; SNAPEDA_LINK: https://www.snapeda.com/parts/BK-18650-PC4/Memory+Protection+Devices/view-part/?ref=snap
C1-C40 = rcl:C-EU: CAPACITOR, European symbol
C41 C44 C47 = rcl:CPOL-EU: POLARIZED CAPACITOR, European symbol
D2 = diode:DIODE-: DIODE
DIS1 = diy-modules:DISPLAY-NOKIA-5110
J1 J2 = con-harting-ml:ML64: HARTING; OC_FARNELL: unknown; OC_NEWARK: unknown
J3 J4 = IDC50PIN:3-1761608-6: IDC LOW PRO HDR 24P VERT SHT L Check availability; AVAILABILITY: In Stock; CENTERLINE_PITCH: 2.54 mm[.1 in]; CHECK_PRICES: https://www.snapeda.com/parts/3-1761608-6/TE+Connectivity/view-part/?ref=eda; COMMENT: 3-1761608-6; DESCRIPTION: Conn Ejector Header HDR 60 POS 2.54mm Solder ST Thru-Hole Tube; EU_ROHS_COMPLIANCE: Compliant; MF: TE Connectivity; MP: 3-1761608-6; NUMBER_OF_POSITIONS: 60; PACKAGE: None; PRICE: None; PRODUCT_TYPE: Connector; SNAPEDA_LINK: https://www.snapeda.com/parts/3-1761608-6/TE+Connectivity/view-part/?ref=snap
J5 J6 = con-harting-ml:ML50: HARTING; OC_FARNELL: unknown; OC_NEWARK: unknown
J7 J8 = con-harting-ml:ML40: HARTING; OC_FARNELL: unknown; OC_NEWARK: unknown
J9 J10 = con-harting-ml:ML34: HARTING; OC_FARNELL: unknown; OC_NEWARK: unknown
J11 J13 = con-ml:ML26: HARTING; OC_FARNELL: unknown; OC_NEWARK: unknown
J12 = con-jack:JACK-PLUG: DC POWER JACK Power Jack, DC, Right Angle, Through Hole, Rated 5A at 16VDC, PC Terminals Distributor: Farnell (www.Farnell.de) Drawing: 84N1161.pdf / 84N1162.pdf Manufacturer: SPC Technology (www.spctechnology.com) Type: SPC4077 / SPC 4078; OC_FARNELL: unknown; OC_NEWARK: unknown
J14 J15 = con-harting-ml:ML20: HARTING; OC_FARNELL: unknown; OC_NEWARK: unknown
J16 J17 = con-harting-ml:ML16: HARTING; OC_FARNELL: unknown; OC_NEWARK: unknown
J18 J19 = con-harting-ml:ML14: HARTING; OC_FARNELL: unknown; OC_NEWARK: unknown
J20-J22 = con-harting-ml:ML10: HARTING; OC_FARNELL: unknown; OC_NEWARK: unknown
JP1 = jumper:JP2E: JUMPER
Q1 = transistor-fet:STR2P3LLH6
Q2 = transistor:BC846: NPN TRANSISTOR
R1-R98 R103-R106 R136-R140 = rcl:R-EU_: RESISTOR, European symbol
RN1-RN12 = resistor-dil:CAY16-J8
SW1-SW3 SW5 SW6 = switch-omron:10-XX: OMRON SWITCH; MPN: B3F-1000; OC_FARNELL: 176432; OC_NEWARK: 36M3542
SW7 = 100DP1T2B4M6QE:100DP1T2B4M6QE: Check availability; AVAILABILITY: In Stock; CHECK_PRICES: https://www.snapeda.com/parts/100DP1T2B4M6QE/E-Switch/view-part/?ref=eda; DESCRIPTION: Toggle Switch, 100 Series, DPDT, ON-NONE-ON, Sealed, 5A, 120VAC, 28VDC, R/A PC | E-Switch 100DP1T2B4M6QE; MF: E-Switch; MP: 100DP1T2B4M6QE; PACKAGE: None; PRICE: None; PURCHASE-URL: https://www.snapeda.com/api/url_track_click_mouser/?unipart_id=2771250&manufacturer=E-Switch&part_name=100DP1T2B4M6QE&search_term=toggle switch dpdt pcb; SNAPEDA_LINK: https://www.snapeda.com/parts/100DP1T2B4M6QE/E-Switch/view-part/?ref=snap
U1-U8 = MCP23017-E_SO:MCP23017-E/SO: MCP23017 Series 5.5 V 1.7 MHz SMT 16-Bit I2C I/O Expander - SOIC-28 Check availability; AVAILABILITY: In Stock; CHECK_PRICES: https://www.snapeda.com/parts/MCP23017-E/SO/Microchip/view-part/?ref=eda; DESCRIPTION: I/O Port Expander, 16-Bit, I2C I'face, SOIC-28 | Microchip Technology Inc. MCP23017-E/SO; MF: Microchip; MP: MCP23017-E/SO; PACKAGE: SOIC-28 Microchip; PRICE: None; PURCHASE-URL: https://www.snapeda.com/api/url_track_click_mouser/?unipart_id=48467&manufacturer=Microchip&part_name=MCP23017-E/SO&search_term=mcp23017; SNAPEDA_LINK: https://www.snapeda.com/parts/MCP23017-E/SO/Microchip/view-part/?ref=snap
U11-U13 = v-reg:LD117A?*: Low drop fixed and adjustable positive voltage regulators 1 A Source: http://www.st.com/stonline/products/literature/ds/7194/ld1117axx.pdf
X2 = con-wago255:234-203: WAGO; MPN: 234-203; OC_FARNELL: unknown; OC_NEWARK: 28K9092
X6 = con-wago255:234-236: WAGO; MPN: 234-236; OC_FARNELL: unknown; OC_NEWARK: 28K9103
